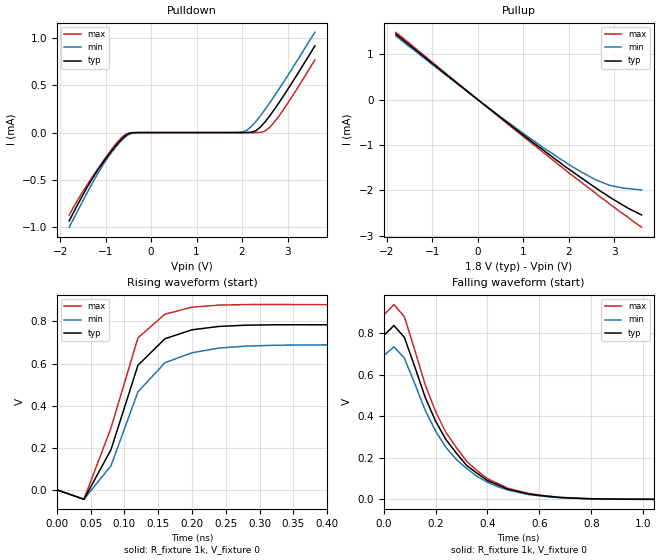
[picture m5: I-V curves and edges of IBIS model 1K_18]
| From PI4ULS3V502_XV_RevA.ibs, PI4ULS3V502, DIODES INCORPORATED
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[Model]   1K_18
Model_type  Output
Vref = 0
Rref = 10k
Vmeas = 0.9
C_comp   8.966pF   8.863pF   9.079pF
[Voltage Range]   1.80V   1.62V   1.98V
[Temperature Range]   25   85   -40
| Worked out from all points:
|   slope of the pullup table from 0 to 0.27 V, typ, clamps not added: 1.27 kohm
|   rising waveform, R_fixture 1k, V_fixture 0: 20-80 % time 56.7ps typ, 61.7ps min, 52.2ps max; typ from 0 V to 0.783 V
|   falling waveform, R_fixture 1k, V_fixture 0: 20-80 % time 203ps typ, 209ps min, 202ps max; typ from 0.789 V to 0 V
[Pullup]
-1.8V     1.44mA     1.4mA      1.48mA
500mV     -393uA     -377uA     -408uA
1.4V      -1.08mA    -1.03mA    -1.13mA
2V        -1.53mA    -1.43mA    -1.61mA
2.5V      -1.88mA    -1.72mA    -1.99mA
2.9V      -2.15mA    -1.89mA    -2.3mA
3.3V      -2.39mA    -1.96mA    -2.59mA
3.6V      -2.54mA    -1.99mA    -2.81mA
[Pulldown]
-1.8V     -934uA     -1mA       -872uA
-1.4V     -574uA     -632uA     -549uA
-1.1V     -346uA     -375uA     -334uA
-600mV    -46.8uA    -60.1uA    -31.2uA
-300mV    -81.3nA    -446nA     -4.46nA
1.9V      263pA      512nA      15pA
2.1V      230nA      23.2uA     26.2pA
2.3V      18.7uA     115uA      51.3nA
2.5V      110uA      240uA      13.8uA
2.6V      171uA      308uA      50.7uA
2.9V      379uA      525uA      236uA
3.6V      916uA      1.06mA     768uA
[Rising Waveform]
R_fixture =   1k
C_fixture =   0
L_fixture =   0
V_fixture =   0
V_fixture_min = 0
V_fixture_max = 0
|   Time   V(typ)   V(min)   V(max)
0s        0V         0V         0V
40ps      -45.07mV   -44.7mV    -44.44mV
80ps      190.2mV    114.2mV    293.2mV
120ps     591.9mV    465.7mV    722.1mV
160ps     718mV      604.1mV    834.7mV
200ps     760.4mV    651.4mV    867.9mV
240ps     776.4mV    673.6mV    877.8mV
280ps     782.3mV    683mV      880.3mV
400ps     784.1mV    688.6mV    879.8mV
3.96ns    783.3mV    687.6mV    879.4mV
[Falling Waveform]
R_fixture =   1k
C_fixture =   0
L_fixture =   0
V_fixture =   0
V_fixture_min = 0
V_fixture_max = 0
|   Time   V(typ)   V(min)   V(max)
0s        788.9mV    691.5mV    887.3mV
40ps      837.8mV    735.2mV    939.4mV
80ps      781mV      680.8mV    880.7mV
160ps     492.1mV    429.1mV    553.5mV
200ps     377mV      328.8mV    423.4mV
320ps     162.4mV    147.9mV    182.4mV
400ps     89.82mV    81.33mV    98.76mV
560ps     24.86mV    21.66mV    26.94mV
920ps     -356.6uV   -557.9uV   -371uV
3.96ns    0V         0V         0V
[Ramp]
| variable   typ   min   max
dV/dt_r   0.5/52.4E-12   0.5/56.8E-12   0.5/46.9E-12
dV/dt_f   0.5/204.2E-12   0.5/209.4E-12   0.5/203.7E-12
R_load = 1k
